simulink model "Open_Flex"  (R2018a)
settings: Solver=VariableStepAuto  StartTime=0.0  StopTime=30  FixedStep=0.0001  RelTol=1e-5  EnableMultiTasking=on
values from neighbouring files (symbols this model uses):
  d2r = pi/180    (= 0.0174532925199)    [init.m]    (also in LQR_Design.m)
  Kr = Kq; Kr(3)=-Kq(3)    [init.m]
  Wf = 18    [init.m]
undefined symbols (not defined in the file or in its folder): Aa, Av, Ba, Bv, Ca, Cv, Da, Dv, Kq, TVC

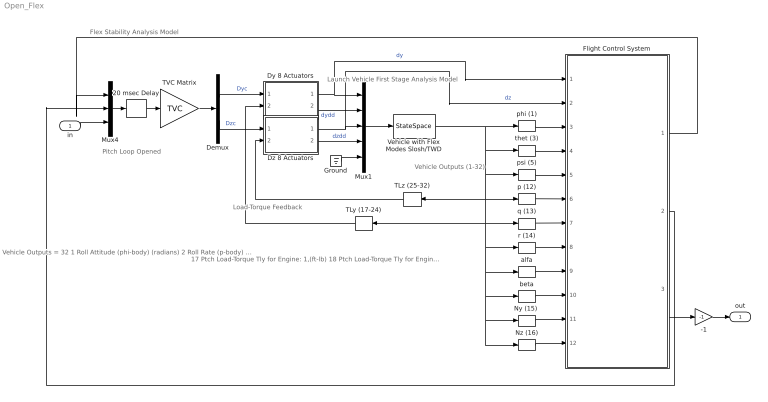
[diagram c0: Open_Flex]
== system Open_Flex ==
  note: Load-Torque Feedback
  note: 17 Ptch Load-Torque Tly for Engine: 1,(ft-lb) 18 Ptch Load-Torque Tly for Engine: 2,(ft-lb) 19 Ptch Load-Torque Tly for Engine: 3,(ft-lb) 20 Ptch Load-Torque Tly for Engine: 4,(ft-lb) 21 Ptch Load-Torque Tly for Engine: 5,(ft-lb) 22 Ptch Load-Torque Tly for Engine: 6,(ft-lb) 23 Ptch Load-Torque Tly for Engine: 7,(ft-lb) 24 Ptch Load-Torque Tly for Engine: 8,(ft-lb) 25 Yaw Load-Torque Tlz for Engine: 1,(ft-lb) 26 Yaw Load-Torque Tlz for Engine: 2,(ft-lb) 27 Yaw Load-Torque Tlz for Engine: 3,(ft-lb) 28 Yaw Load-Torque Tlz for Engine: 4,(ft-lb) 29 Yaw Load-Torque Tlz for Engine: 5,(ft-lb) 30 Yaw Load-Torque Tlz for Engine: 6,(ft-lb) 31 Yaw Load-Torque Tlz for Engine: 7,(ft-lb) 32 Yaw Load-Torque Tlz for Engine: 8,(ft-lb)
  note: Vehicle Outputs = 32 1 Roll Attitude (phi-body) (radians) 2 Roll Rate (p-body) (rad/sec) 3 Pitch Attitude (thet-bdy) (radians) 4 Pitch Rate (q-body) (rad/sec) 5 Yaw Attitude (psi-body) (radians) 6 Yaw Rate (r-body) (rad/sec) 7 Angle of attack, alfa, (radians) 8 Angle of sideslip, beta, (radian) 9 Change in Altitude, delta-h, (feet) 10 Forward Acceleration (V-dot) (ft/sec) 11 Cross Range Velocity (Vcr) (ft/sec) 12 Rate-Gyro # 1, Roll Rate (Body) (rad/sec) 13 Rate-Gyro # 2, Pitch Rate (Body) (rad/sec) 14 Rate-Gyro # 3, Yaw Rate (Body) (rad/sec) 15 Accelerom # 1, (along Y), (ft/sec^2) Translat. Accelerat. 16 Accelerom # 2, (along Z), (ft/sec^2) Translat. Accelerat.
  note: Vehicle Outputs (1-32)
  note: Launch Vehicle First Stage Analysis Model
  note: Flex Stability Analysis Model
  note: Pitch Loop Opened
  in : Inport
  -1 : Gain  Gain=-1
  20 msec Delay : TransportDelay  DelayTime="[1  1  1]*0.02"  InitialOutput="[0  0  0]"  PadeOrder=2
  Demux : Demux  Outputs=[8, 8]
  Dy 8 Actuators : Subsystem
  Dz 8 Actuators : Subsystem
  Flight Control System : Subsystem
  Ground : Ground
  Mux1 : Mux  Inputs=[8, 8, 8, 8, 1]
  Mux4 : Mux  Inputs=3
  "Ny (15) " : Selector  InputPortWidth=32  IndexOptions=Index vector (dialog)  Indices=[15]  OutputSizes=1
  Nz (16) : Selector  InputPortWidth=32  IndexOptions=Index vector (dialog)  Indices=[16]  OutputSizes=1
  TLy (17-24) : Selector  InputPortWidth=32  IndexOptions=Index vector (dialog)  Indices=[17:24]  OutputSizes=1
  TLz (25-32) : Selector  InputPortWidth=32  IndexOptions=Index vector (dialog)  Indices=[25:32]  OutputSizes=1
  TVC Matrix : Gain  Gain=TVC  Multiplication=Matrix(K*u)
  Vehicle with Flex Modes Slosh/TWD : StateSpace  A=Av  B=Bv  C=Cv  D=Dv  InitialCondition=0
  alfa : Selector  InputPortWidth=32  IndexOptions=Index vector (dialog)  Indices=[7]  OutputSizes=1
  beta : Selector  InputPortWidth=32  IndexOptions=Index vector (dialog)  Indices=[8]  OutputSizes=1
  p (12) : Selector  InputPortWidth=32  IndexOptions=Index vector (dialog)  Indices=[12]  OutputSizes=1
  phi (1) : Selector  InputPortWidth=32  IndexOptions=Index vector (dialog)  Indices=[1]  OutputSizes=1
  psi (5) : Selector  InputPortWidth=32  IndexOptions=Index vector (dialog)  Indices=[5]  OutputSizes=1
  q (13) : Selector  InputPortWidth=32  IndexOptions=Index vector (dialog)  Indices=[13]  OutputSizes=1
  r (14) : Selector  InputPortWidth=32  IndexOptions=Index vector (dialog)  Indices=[14]  OutputSizes=1
  thet (3) : Selector  InputPortWidth=32  IndexOptions=Index vector (dialog)  Indices=[3]  OutputSizes=1
  out : Outport
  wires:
  Mux1/1 -> Vehicle with Flex Modes Slosh/TWD/1
  Dy 8 Actuators/2(dydd) -> Mux1/2  "dydd"
  Dz 8 Actuators/2(dzdd) -> Mux1/4  "dzdd"
  Demux/1 -> Dy 8 Actuators/1(dyc)  "Dyc"
  Dy 8 Actuators/1(dy) -> Flight Control System/1(dy), Mux1/1  "dy"
  Dz 8 Actuators/1(dz) -> Flight Control System/2(dz), Mux1/3  "dz"
  Demux/2 -> Dz 8 Actuators/1(dzc)  "Dzc"
  TLy (17-24)/1 -> Dy 8 Actuators/2(TLy)
  TLz (25-32)/1 -> Dz 8 Actuators/2(TLz)
  Mux4/1 -> 20 msec Delay/1
  TVC Matrix/1 -> Demux/1
  -1/1 -> out/1
  Ground/1 -> Mux1/5
  Vehicle with Flex Modes Slosh/TWD/1 -> thet (3)/1, psi (5)/1, Nz (16)/1, "Ny (15) "/1, beta/1, alfa/1, r (14)/1, TLy (17-24)/1, q (13)/1, TLz (25-32)/1, p (12)/1, phi (1)/1
  Nz (16)/1 -> Flight Control System/12(NZ)
  "Ny (15) "/1 -> Flight Control System/11(NY)
  beta/1 -> Flight Control System/10(beta)
  alfa/1 -> Flight Control System/9(alfa)
  r (14)/1 -> Flight Control System/8(r)
  q (13)/1 -> Flight Control System/7(q)
  p (12)/1 -> Flight Control System/6(p)
  psi (5)/1 -> Flight Control System/5(psi)
  thet (3)/1 -> Flight Control System/4(thet)
  phi (1)/1 -> Flight Control System/3(phi)
  20 msec Delay/1 -> TVC Matrix/1
  Flight Control System/1(DP_tvc) -> Mux4/1
  in/1 -> Mux4/3
  Flight Control System/3(DR_tvc) -> -1/1
  Flight Control System/2(DQ_tvc) -> Mux4/2

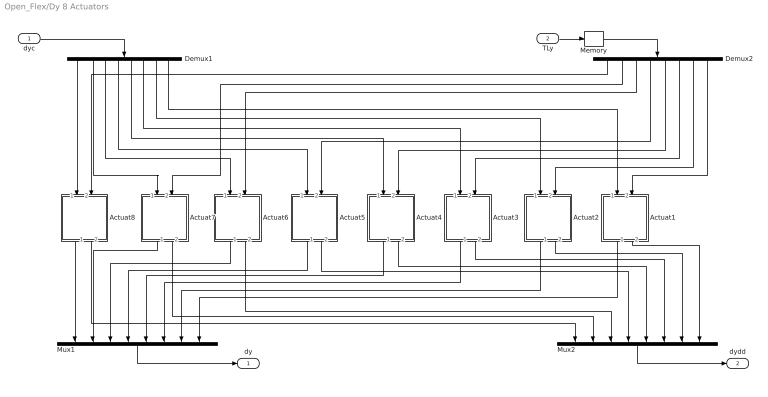
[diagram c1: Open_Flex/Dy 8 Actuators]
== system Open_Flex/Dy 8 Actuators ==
  dyc : Inport
  TLy : Inport  Port=2
  Actuat1 : Subsystem
  Actuat2 : Subsystem
  Actuat3 : Subsystem
  Actuat4 : Subsystem
  Actuat5 : Subsystem
  Actuat6 : Subsystem
  Actuat7 : Subsystem
  Actuat8 : Subsystem
  Demux1 : Demux  Outputs=8
  Demux2 : Demux  Outputs=8
  Memory : Memory  LinearizeAsDelay=on
  Mux1 : Mux  Inputs=8
  Mux2 : Mux  Inputs=8
  dy : Outport
  dydd : Outport  Port=2
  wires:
  TLy/1 -> Memory/1
  Mux2/1 -> dydd/1
  Actuat5/1(dout) -> Mux1/4
  Demux1/5 -> Actuat4/1(delin)
  Actuat3/2(ddot) -> Mux2/6
  Actuat8/1(dout) -> Mux1/1
  Demux1/4 -> Actuat5/1(delin)
  Actuat1/1(dout) -> Mux1/8
  Actuat4/2(ddot) -> Mux2/5
  Actuat4/1(dout) -> Mux1/5
  Demux2/4 -> Actuat5/2(TL)
  Demux2/6 -> Actuat3/2(TL)
  Demux2/7 -> Actuat2/2(TL)
  Actuat6/2(ddot) -> Mux2/3
  Demux2/2 -> Actuat7/2(TL)
  Actuat5/2(ddot) -> Mux2/4
  Demux1/3 -> Actuat6/1(delin)
  Actuat2/2(ddot) -> Mux2/7
  Actuat8/2(ddot) -> Mux2/1
  dyc/1 -> Demux1/1
  Mux1/1 -> dy/1
  Actuat1/2(ddot) -> Mux2/8
  Actuat7/2(ddot) -> Mux2/2
  Demux1/2 -> Actuat7/1(delin)
  Demux1/7 -> Actuat2/1(delin)
  Demux1/8 -> Actuat1/1(delin)
  Actuat7/1(dout) -> Mux1/2
  Demux2/5 -> Actuat4/2(TL)
  Demux1/1 -> Actuat8/1(delin)
  Demux2/1 -> Actuat8/2(TL)
  Actuat2/1(dout) -> Mux1/7
  Demux2/8 -> Actuat1/2(TL)
  Demux2/3 -> Actuat6/2(TL)
  Actuat3/1(dout) -> Mux1/6
  Actuat6/1(dout) -> Mux1/3
  Demux1/6 -> Actuat3/1(delin)
  Memory/1 -> Demux2/1

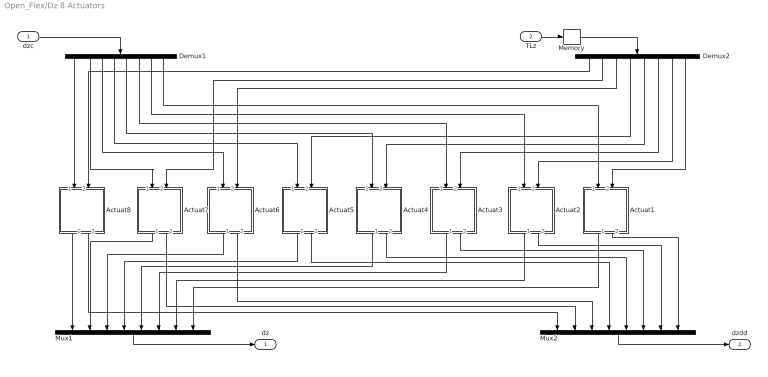
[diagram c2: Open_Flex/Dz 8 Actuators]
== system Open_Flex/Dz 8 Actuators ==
  dzc : Inport
  TLz : Inport  Port=2
  Actuat1 : Subsystem
  Actuat2 : Subsystem
  Actuat3 : Subsystem
  Actuat4 : Subsystem
  Actuat5 : Subsystem
  Actuat6 : Subsystem
  Actuat7 : Subsystem
  Actuat8 : Subsystem
  Demux1 : Demux  Outputs=8
  Demux2 : Demux  Outputs=8
  Memory : Memory  LinearizeAsDelay=on
  Mux1 : Mux  Inputs=8
  Mux2 : Mux  Inputs=8
  dz : Outport
  dzdd : Outport  Port=2
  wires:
  TLz/1 -> Memory/1
  Mux2/1 -> dzdd/1
  Actuat5/1(dout) -> Mux1/4
  Demux1/5 -> Actuat4/1(delin)
  Actuat3/2(ddot) -> Mux2/6
  Actuat8/1(dout) -> Mux1/1
  Demux1/4 -> Actuat5/1(delin)
  Actuat1/1(dout) -> Mux1/8
  Actuat4/2(ddot) -> Mux2/5
  Actuat4/1(dout) -> Mux1/5
  Demux2/4 -> Actuat5/2(TL)
  Demux2/6 -> Actuat3/2(TL)
  Demux2/7 -> Actuat2/2(TL)
  Actuat6/2(ddot) -> Mux2/3
  Demux2/2 -> Actuat7/2(TL)
  Actuat5/2(ddot) -> Mux2/4
  Demux1/3 -> Actuat6/1(delin)
  Actuat2/2(ddot) -> Mux2/7
  Actuat8/2(ddot) -> Mux2/1
  dzc/1 -> Demux1/1
  Mux1/1 -> dz/1
  Actuat1/2(ddot) -> Mux2/8
  Actuat7/2(ddot) -> Mux2/2
  Demux1/2 -> Actuat7/1(delin)
  Demux1/7 -> Actuat2/1(delin)
  Demux1/8 -> Actuat1/1(delin)
  Actuat7/1(dout) -> Mux1/2
  Demux2/5 -> Actuat4/2(TL)
  Demux1/1 -> Actuat8/1(delin)
  Demux2/1 -> Actuat8/2(TL)
  Actuat2/1(dout) -> Mux1/7
  Demux2/8 -> Actuat1/2(TL)
  Demux2/3 -> Actuat6/2(TL)
  Actuat3/1(dout) -> Mux1/6
  Actuat6/1(dout) -> Mux1/3
  Demux1/6 -> Actuat3/1(delin)
  Memory/1 -> Demux2/1

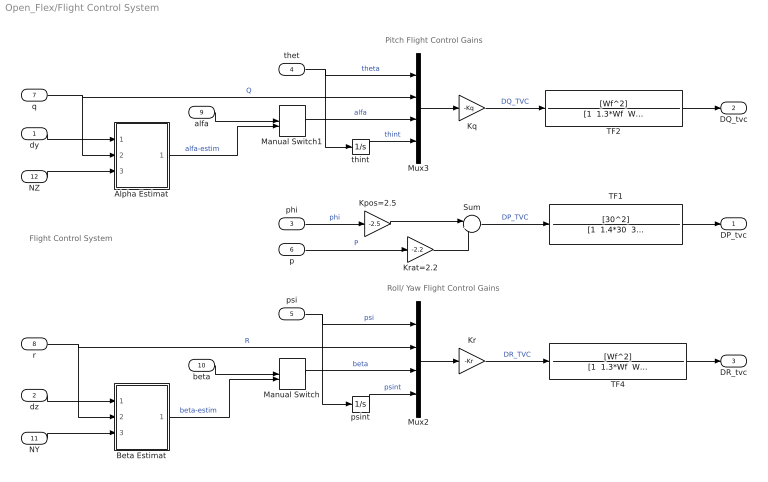
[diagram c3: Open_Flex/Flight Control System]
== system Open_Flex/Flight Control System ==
  note: Flight Control System
  note: Roll/ Yaw Flight Control Gains
  note: Pitch Flight Control Gains
  dy : Inport
  dz : Inport  Port=2
  phi : Inport  Port=3
  thet : Inport  Port=4
  psi : Inport  Port=5
  p : Inport  Port=6
  q : Inport  Port=7
  r : Inport  Port=8
  alfa : Inport  Port=9
  beta : Inport  Port=10
  NY : Inport  Port=11
  NZ : Inport  Port=12
  Alpha Estimat : Subsystem
  Beta Estimat : Subsystem
  Kpos=2.5 : Gain  Gain=-2.5  Multiplication=Matrix(K*u)
  Kq : Gain  Gain=-Kq  Multiplication=Matrix(K*u)
  Kr : Gain  Gain=-Kr  Multiplication=Matrix(K*u)
  Krat=2.2 : Gain  Gain=-2.2  Multiplication=Matrix(K*u)
  Manual Switch : ManualSwitch  CurrentSetting=0
  Manual Switch1 : ManualSwitch  CurrentSetting=0
  Mux2 : Mux
  Mux3 : Mux
  Sum : Sum  Inputs=|++
  TF1 : TransferFcn  Numerator=[30^2]  Denominator="[1  1.4*30  30^2]"
  TF2 : TransferFcn  Numerator=[Wf^2]  Denominator="[1  1.3*Wf  Wf^2]"
  TF4 : TransferFcn  Numerator=[Wf^2]  Denominator="[1  1.3*Wf  Wf^2]"
  psint : Integrator
  thint : Integrator
  DP_tvc : Outport
  DQ_tvc : Outport  Port=2
  DR_tvc : Outport  Port=3
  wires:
  TF1/1 -> DP_tvc/1
  Mux2/1 -> Kr/1
  phi/1 -> Kpos=2.5/1  "phi"
  p/1 -> Krat=2.2/1  "P"
  Krat=2.2/1 -> Sum/2
  Sum/1 -> TF1/1  "DP_TVC"
  Kpos=2.5/1 -> Sum/1
  Mux3/1 -> Kq/1
  dz/1 -> Beta Estimat/1(dz)
  dy/1 -> Alpha Estimat/1(dy)
  Beta Estimat/1(betest) -> Manual Switch/2  "beta-estim"
  NY/1 -> Beta Estimat/3(Ydd)
  NZ/1 -> Alpha Estimat/3(Zdd)
  TF2/1 -> DQ_tvc/1
  TF4/1 -> DR_tvc/1
  Kq/1 -> TF2/1  "DQ_TVC"
  thet/1 -> Mux3/1, thint/1  "theta"
  Kr/1 -> TF4/1  "DR_TVC"
  thint/1 -> Mux3/4  "thint"
  r/1 -> Mux2/2, Beta Estimat/2(r)  "R"
  q/1 -> Mux3/2, Alpha Estimat/2(q)  "Q"
  psint/1 -> Mux2/4  "psint"
  psi/1 -> Mux2/1, psint/1  "psi"
  Manual Switch/1 -> Mux2/3  "beta"
  beta/1 -> Manual Switch/1
  Manual Switch1/1 -> Mux3/3  "alfa"
  alfa/1 -> Manual Switch1/1
  Alpha Estimat/1(alfest) -> Manual Switch1/2  "alfa-estim"

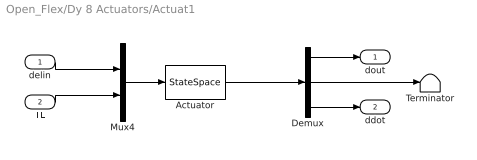
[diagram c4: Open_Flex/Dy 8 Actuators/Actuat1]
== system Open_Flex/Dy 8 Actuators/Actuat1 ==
  delin : Inport
  TL : Inport  Port=2
  Actuator : StateSpace  A=Aa  B=Ba  C=Ca  D=Da  InitialCondition=0
  Demux : Demux  Outputs=3
  Mux4 : Mux  Inputs=2
  Terminator : Terminator
  dout : Outport
  ddot : Outport  Port=2
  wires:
  Demux/3 -> ddot/1
  TL/1 -> Mux4/2
  Mux4/1 -> Actuator/1
  Actuator/1 -> Demux/1
  delin/1 -> Mux4/1
  Demux/1 -> dout/1
  Demux/2 -> Terminator/1

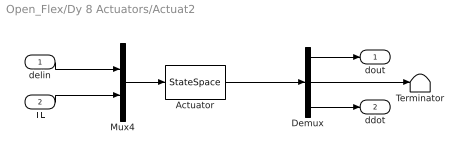
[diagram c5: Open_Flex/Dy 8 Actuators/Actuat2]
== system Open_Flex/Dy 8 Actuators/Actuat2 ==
  delin : Inport
  TL : Inport  Port=2
  Actuator : StateSpace  A=Aa  B=Ba  C=Ca  D=Da  InitialCondition=0
  Demux : Demux  Outputs=3
  Mux4 : Mux  Inputs=2
  Terminator : Terminator
  dout : Outport
  ddot : Outport  Port=2
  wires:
  Demux/3 -> ddot/1
  TL/1 -> Mux4/2
  Mux4/1 -> Actuator/1
  Actuator/1 -> Demux/1
  delin/1 -> Mux4/1
  Demux/1 -> dout/1
  Demux/2 -> Terminator/1

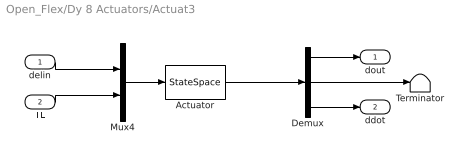
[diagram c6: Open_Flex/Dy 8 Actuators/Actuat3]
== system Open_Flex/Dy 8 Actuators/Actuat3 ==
  delin : Inport
  TL : Inport  Port=2
  Actuator : StateSpace  A=Aa  B=Ba  C=Ca  D=Da  InitialCondition=0
  Demux : Demux  Outputs=3
  Mux4 : Mux  Inputs=2
  Terminator : Terminator
  dout : Outport
  ddot : Outport  Port=2
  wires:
  Demux/3 -> ddot/1
  TL/1 -> Mux4/2
  Mux4/1 -> Actuator/1
  Actuator/1 -> Demux/1
  delin/1 -> Mux4/1
  Demux/1 -> dout/1
  Demux/2 -> Terminator/1

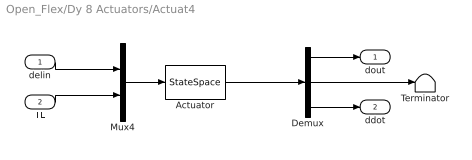
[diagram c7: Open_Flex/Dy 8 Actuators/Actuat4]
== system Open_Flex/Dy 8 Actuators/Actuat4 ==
  delin : Inport
  TL : Inport  Port=2
  Actuator : StateSpace  A=Aa  B=Ba  C=Ca  D=Da  InitialCondition=0
  Demux : Demux  Outputs=3
  Mux4 : Mux  Inputs=2
  Terminator : Terminator
  dout : Outport
  ddot : Outport  Port=2
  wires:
  Demux/3 -> ddot/1
  TL/1 -> Mux4/2
  Mux4/1 -> Actuator/1
  Actuator/1 -> Demux/1
  delin/1 -> Mux4/1
  Demux/1 -> dout/1
  Demux/2 -> Terminator/1

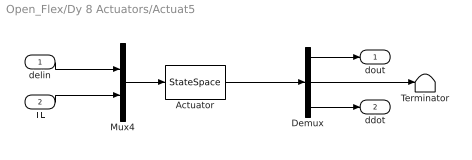
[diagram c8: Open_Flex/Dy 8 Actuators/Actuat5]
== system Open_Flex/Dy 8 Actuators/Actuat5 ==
  delin : Inport
  TL : Inport  Port=2
  Actuator : StateSpace  A=Aa  B=Ba  C=Ca  D=Da  InitialCondition=0
  Demux : Demux  Outputs=3
  Mux4 : Mux  Inputs=2
  Terminator : Terminator
  dout : Outport
  ddot : Outport  Port=2
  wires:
  Demux/3 -> ddot/1
  TL/1 -> Mux4/2
  Mux4/1 -> Actuator/1
  Actuator/1 -> Demux/1
  delin/1 -> Mux4/1
  Demux/1 -> dout/1
  Demux/2 -> Terminator/1

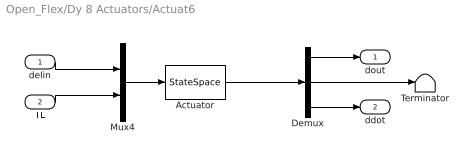
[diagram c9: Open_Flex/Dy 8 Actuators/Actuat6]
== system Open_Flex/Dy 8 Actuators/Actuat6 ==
  delin : Inport
  TL : Inport  Port=2
  Actuator : StateSpace  A=Aa  B=Ba  C=Ca  D=Da  InitialCondition=0
  Demux : Demux  Outputs=3
  Mux4 : Mux  Inputs=2
  Terminator : Terminator
  dout : Outport
  ddot : Outport  Port=2
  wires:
  Demux/3 -> ddot/1
  TL/1 -> Mux4/2
  Mux4/1 -> Actuator/1
  Actuator/1 -> Demux/1
  delin/1 -> Mux4/1
  Demux/1 -> dout/1
  Demux/2 -> Terminator/1

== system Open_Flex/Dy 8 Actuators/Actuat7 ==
  delin : Inport
  TL : Inport  Port=2
  Actuator : StateSpace  A=Aa  B=Ba  C=Ca  D=Da  InitialCondition=0
  Demux : Demux  Outputs=3
  Mux4 : Mux  Inputs=2
  Terminator : Terminator
  dout : Outport
  ddot : Outport  Port=2
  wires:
  Demux/3 -> ddot/1
  TL/1 -> Mux4/2
  Mux4/1 -> Actuator/1
  Actuator/1 -> Demux/1
  delin/1 -> Mux4/1
  Demux/1 -> dout/1
  Demux/2 -> Terminator/1

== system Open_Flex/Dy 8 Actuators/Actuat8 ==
  delin : Inport
  TL : Inport  Port=2
  Actuator : StateSpace  A=Aa  B=Ba  C=Ca  D=Da  InitialCondition=0
  Demux : Demux  Outputs=3
  Mux4 : Mux  Inputs=2
  Terminator : Terminator
  dout : Outport
  ddot : Outport  Port=2
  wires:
  Demux/3 -> ddot/1
  TL/1 -> Mux4/2
  Mux4/1 -> Actuator/1
  Actuator/1 -> Demux/1
  delin/1 -> Mux4/1
  Demux/1 -> dout/1
  Demux/2 -> Terminator/1

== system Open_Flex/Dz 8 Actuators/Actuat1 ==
  delin : Inport
  TL : Inport  Port=2
  Actuator : StateSpace  A=Aa  B=Ba  C=Ca  D=Da  InitialCondition=0
  Demux : Demux  Outputs=3
  Mux4 : Mux  Inputs=2
  Terminator : Terminator
  dout : Outport
  ddot : Outport  Port=2
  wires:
  Demux/3 -> ddot/1
  TL/1 -> Mux4/2
  Mux4/1 -> Actuator/1
  Actuator/1 -> Demux/1
  delin/1 -> Mux4/1
  Demux/1 -> dout/1
  Demux/2 -> Terminator/1

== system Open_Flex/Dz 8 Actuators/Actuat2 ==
  delin : Inport
  TL : Inport  Port=2
  Actuator : StateSpace  A=Aa  B=Ba  C=Ca  D=Da  InitialCondition=0
  Demux : Demux  Outputs=3
  Mux4 : Mux  Inputs=2
  Terminator : Terminator
  dout : Outport
  ddot : Outport  Port=2
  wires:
  Demux/3 -> ddot/1
  TL/1 -> Mux4/2
  Mux4/1 -> Actuator/1
  Actuator/1 -> Demux/1
  delin/1 -> Mux4/1
  Demux/1 -> dout/1
  Demux/2 -> Terminator/1

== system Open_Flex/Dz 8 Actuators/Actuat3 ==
  delin : Inport
  TL : Inport  Port=2
  Actuator : StateSpace  A=Aa  B=Ba  C=Ca  D=Da  InitialCondition=0
  Demux : Demux  Outputs=3
  Mux4 : Mux  Inputs=2
  Terminator : Terminator
  dout : Outport
  ddot : Outport  Port=2
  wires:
  Demux/3 -> ddot/1
  TL/1 -> Mux4/2
  Mux4/1 -> Actuator/1
  Actuator/1 -> Demux/1
  delin/1 -> Mux4/1
  Demux/1 -> dout/1
  Demux/2 -> Terminator/1

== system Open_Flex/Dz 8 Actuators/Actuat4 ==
  delin : Inport
  TL : Inport  Port=2
  Actuator : StateSpace  A=Aa  B=Ba  C=Ca  D=Da  InitialCondition=0
  Demux : Demux  Outputs=3
  Mux4 : Mux  Inputs=2
  Terminator : Terminator
  dout : Outport
  ddot : Outport  Port=2
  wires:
  Demux/3 -> ddot/1
  TL/1 -> Mux4/2
  Mux4/1 -> Actuator/1
  Actuator/1 -> Demux/1
  delin/1 -> Mux4/1
  Demux/1 -> dout/1
  Demux/2 -> Terminator/1

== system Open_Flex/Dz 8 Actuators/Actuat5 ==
  delin : Inport
  TL : Inport  Port=2
  Actuator : StateSpace  A=Aa  B=Ba  C=Ca  D=Da  InitialCondition=0
  Demux : Demux  Outputs=3
  Mux4 : Mux  Inputs=2
  Terminator : Terminator
  dout : Outport
  ddot : Outport  Port=2
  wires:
  Demux/3 -> ddot/1
  TL/1 -> Mux4/2
  Mux4/1 -> Actuator/1
  Actuator/1 -> Demux/1
  delin/1 -> Mux4/1
  Demux/1 -> dout/1
  Demux/2 -> Terminator/1

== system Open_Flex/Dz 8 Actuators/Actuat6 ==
  delin : Inport
  TL : Inport  Port=2
  Actuator : StateSpace  A=Aa  B=Ba  C=Ca  D=Da  InitialCondition=0
  Demux : Demux  Outputs=3
  Mux4 : Mux  Inputs=2
  Terminator : Terminator
  dout : Outport
  ddot : Outport  Port=2
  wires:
  Demux/3 -> ddot/1
  TL/1 -> Mux4/2
  Mux4/1 -> Actuator/1
  Actuator/1 -> Demux/1
  delin/1 -> Mux4/1
  Demux/1 -> dout/1
  Demux/2 -> Terminator/1

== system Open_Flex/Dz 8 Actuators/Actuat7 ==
  delin : Inport
  TL : Inport  Port=2
  Actuator : StateSpace  A=Aa  B=Ba  C=Ca  D=Da  InitialCondition=0
  Demux : Demux  Outputs=3
  Mux4 : Mux  Inputs=2
  Terminator : Terminator
  dout : Outport
  ddot : Outport  Port=2
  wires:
  Demux/3 -> ddot/1
  TL/1 -> Mux4/2
  Mux4/1 -> Actuator/1
  Actuator/1 -> Demux/1
  delin/1 -> Mux4/1
  Demux/1 -> dout/1
  Demux/2 -> Terminator/1

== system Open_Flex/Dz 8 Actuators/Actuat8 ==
  delin : Inport
  TL : Inport  Port=2
  Actuator : StateSpace  A=Aa  B=Ba  C=Ca  D=Da  InitialCondition=0
  Demux : Demux  Outputs=3
  Mux4 : Mux  Inputs=2
  Terminator : Terminator
  dout : Outport
  ddot : Outport  Port=2
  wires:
  Demux/3 -> ddot/1
  TL/1 -> Mux4/2
  Mux4/1 -> Actuator/1
  Actuator/1 -> Demux/1
  delin/1 -> Mux4/1
  Demux/1 -> dout/1
  Demux/2 -> Terminator/1

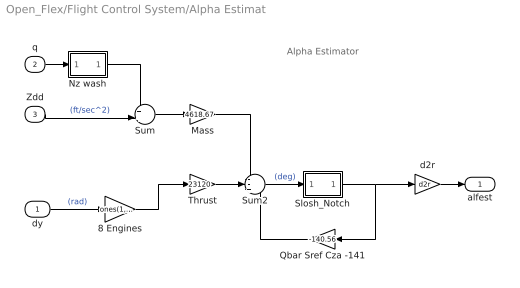
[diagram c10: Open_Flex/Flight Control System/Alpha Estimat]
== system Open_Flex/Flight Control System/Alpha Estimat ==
  note: Alpha Estimator
  dy : Inport
  q : Inport  Port=2
  Zdd : Inport  Port=3
  8 Engines : Gain  Gain=ones(1,8)  Multiplication=Matrix(K*u) (u vector)
  Mass : Gain  Gain=4618.67
  Nz wash : Subsystem
  Qbar Sref Cza -141 : Gain  Gain=-140.56
  Slosh_Notch : Subsystem
  Sum : Sum  Inputs=++|
  Sum2 : Sum  Inputs=--+
  Thrust : Gain  Gain=23120
  d2r : Gain  Gain=d2r
  alfest : Outport
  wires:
  Thrust/1 -> Sum2/2
  dy/1 -> 8 Engines/1  "(rad)"
  Sum/1 -> Mass/1
  q/1 -> Nz wash/1(in)
  d2r/1 -> alfest/1
  Zdd/1 -> Sum/2  "(ft/sec^2)"
  Qbar Sref Cza -141/1 -> Sum2/3
  Sum2/1 -> Slosh_Notch/1(in)  "(deg)"
  Nz wash/1(ou) -> Sum/1
  Slosh_Notch/1(ou) -> d2r/1, Qbar Sref Cza -141/1
  Mass/1 -> Sum2/1
  8 Engines/1 -> Thrust/1

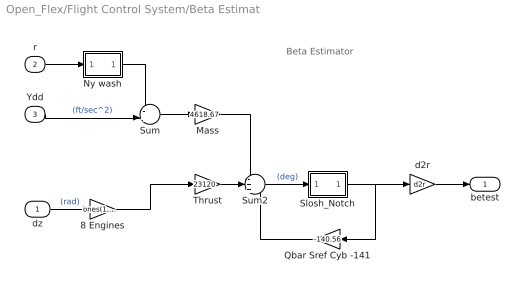
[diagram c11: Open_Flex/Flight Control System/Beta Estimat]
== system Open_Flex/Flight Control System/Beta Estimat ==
  note: Beta Estimator
  dz : Inport
  r : Inport  Port=2
  Ydd : Inport  Port=3
  8 Engines : Gain  Gain=ones(1,8)  Multiplication=Matrix(K*u) (u vector)
  Mass : Gain  Gain=4618.67
  Ny wash : Subsystem
  Qbar Sref Cyb -141 : Gain  Gain=-140.56
  Slosh_Notch : Subsystem
  Sum : Sum  Inputs=-+|
  Sum2 : Sum  Inputs=-++
  Thrust : Gain  Gain=23120
  d2r : Gain  Gain=d2r
  betest : Outport
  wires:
  Sum/1 -> Mass/1
  r/1 -> Ny wash/1(in)
  Thrust/1 -> Sum2/2
  d2r/1 -> betest/1
  Mass/1 -> Sum2/1
  Ydd/1 -> Sum/2  "(ft/sec^2)"
  Qbar Sref Cyb -141/1 -> Sum2/3
  Sum2/1 -> Slosh_Notch/1(in)  "(deg)"
  Ny wash/1(ou) -> Sum/1
  Slosh_Notch/1(ou) -> Qbar Sref Cyb -141/1, d2r/1
  dz/1 -> 8 Engines/1  "(rad)"
  8 Engines/1 -> Thrust/1

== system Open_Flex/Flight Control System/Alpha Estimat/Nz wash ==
  in : Inport
  3 : Gain  Gain=20
  Transfer Fcn : TransferFcn  Numerator="[1  0]"  Denominator="[0.015  1]"
  ou : Outport
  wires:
  in/1 -> Transfer Fcn/1
  Transfer Fcn/1 -> 3/1
  3/1 -> ou/1

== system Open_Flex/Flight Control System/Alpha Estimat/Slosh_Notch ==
  in : Inport
  0.1 : Gain  Gain=0.0015
  Int1 : Integrator
  Transfer Fcn1 : TransferFcn  Numerator="[1 0.016*4  3.72^2]"  Denominator="[1  0.32*4  3.72^2]"
  ou : Outport
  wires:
  in/1 -> 0.1/1
  Int1/1 -> ou/1
  0.1/1 -> Transfer Fcn1/1
  Transfer Fcn1/1 -> Int1/1

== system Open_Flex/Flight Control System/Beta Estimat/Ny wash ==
  in : Inport
  3 : Gain  Gain=20
  Transfer Fcn1 : TransferFcn  Numerator="[1  0]"  Denominator="[0.015  1]"
  ou : Outport
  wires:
  in/1 -> Transfer Fcn1/1
  Transfer Fcn1/1 -> 3/1
  3/1 -> ou/1

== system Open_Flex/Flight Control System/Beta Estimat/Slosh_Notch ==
  in : Inport
  0.0015 : Gain  Gain=0.0015
  Int1 : Integrator
  Transfer Fcn1 : TransferFcn  Numerator="[1 0.016*4  3.72^2]"  Denominator="[1  0.32*4  3.72^2]"
  ou : Outport
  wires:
  in/1 -> 0.0015/1
  Int1/1 -> ou/1
  0.0015/1 -> Transfer Fcn1/1
  Transfer Fcn1/1 -> Int1/1
